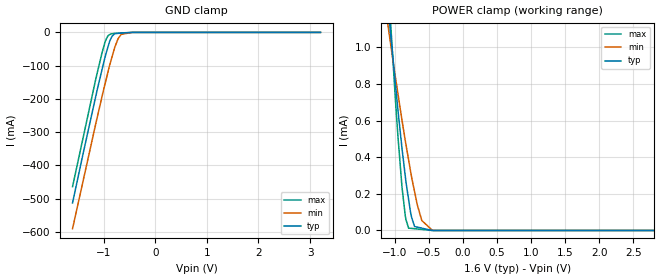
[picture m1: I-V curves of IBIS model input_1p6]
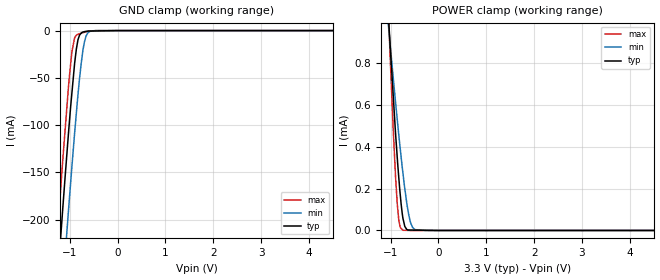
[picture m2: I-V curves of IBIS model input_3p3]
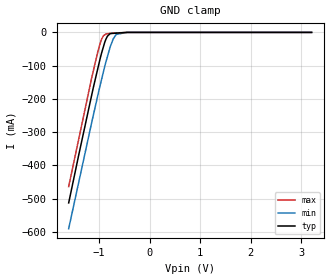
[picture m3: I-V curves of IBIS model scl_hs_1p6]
|Texas Instruments Incorporated
|Low-Power Digital Temperature Sensor with Two-Wire Interface in WCSP
| Marketing part#   Digital Voltage Range   Package-type   #pins
| TMP108YFF   1.4V - 3.6V   WCSP   6
[IBIS Ver]   4.1
[File name]   tmp108.ibs
[File Rev]   1.0
[Date]   12/13/2012
[Source]
| Texas Instruments Incorporated.
| Analog-eLab Design Center, HPA
| 12500 TI Blvd
| Dallas, TX -75243
| e-mail: elab_scm_ibis@list.ti.com
[Notes]   Revision History:
| Rev 1.0: 12/13/2012
| - Initial version of the model
| - Model generated from simulations in TISPICE
| - Model matched to SPICE simulation
| - C_comp although listed in numerical order of value are
|   obtained from varying PVT conditions. For PVT conditions for
|   each specific value refer the buffer description under
|   respective [Model]. IBIS model user is responsible for using
|   appropriate C_comp to simulate for Signal Integrity.
| - Model names with a trailing _1p6 containsthe model for 1.6V
|   [1.4V and 1.8V].Model names with a trailing _3p3 contains the
|   model for 3.3V [3.0V and 3.6V].
[Disclaimer]
| This model is designed as an aid for customers of Texas Instruments.
| TI and its licensors and suppliers make no warranties, either expressed
| or implied, with respect to this  model, including the warranties of
| merchantability or fitness for a particular purpose. The model is
| provided solely on an "as is" basis. The entire risk as to its quality
| and performance is with the customer.
[Copyright]
(C) Copyright 2012 Texas Instruments Incorporated.All rights reserved.
|   TMP108
[Component]   TMP108
[Manufacturer]   TI
[Package]   |6-WCSP
|   typ   min   max
R_pkg   0.00500   0.00500   0.00500
L_pkg   0.20000nH   0.20000nH   0.20000nH
C_pkg   0.60000pF   0.60000pF   0.60000pF
[Pin]  signal_name   model_name   R_pin   L_pin   C_pin
A1   V+   POWER   0.00500   0.20000nH  0.60000pF
A2   GND   GND   0.00500   0.20000nH  0.60000pF
B1   A0   INPUT   0.00500   0.20000nH  0.60000pF
B2   SCL   SCL   0.00500   0.20000nH  0.60000pF
C1   ALERT   ALERT   0.00500   0.20000nH  0.60000pF
C2   SDA   SDA   0.00500   0.20000nH  0.60000pF
|   Model Selectors
[Model Selector] INPUT
input_1p6  1.6V digital input
input_3p3  3.3V digital input
[Model Selector] SCL
scl_hs_1p6  1.6V digital input freq = 2.75MHz
scl_hs_3p3  3.3V digital input freq = 3.4MHz
[Model Selector] ALERT
alert_1p6  1.6V digital open-drain
alert_3p3  3.3V digital open-drain
[Model Selector] SDA
sda_fs_1p6  1.6V digital I/O_open-drain Fast_Speed freq =400KHz
sda_hs_1p6  1.6V digital I/O_open-drain High_Speed freq =3.4MHz
sda_fs_3p3  3.3V digital I/O_open-drain Fast_Speed freq =400KHz
sda_hs_3p3  3.3V digital I/O_open-drain High_Speed freq =3.4MHz
| Models and submodels in the file (10): input_1p6 (Input), input_3p3 (Input), scl_hs_1p6 (Input), scl_hs_3p3 (Input), alert_1p6 (Open_drain), alert_3p3 (Open_drain), sda_fs_1p6 (I/O_open_drain), sda_fs_3p3 (I/O_open_drain), sda_hs_1p6 (I/O_open_drain), sda_hs_3p3 (I/O_open_drain)
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|   input_1p6 Model
[Model]   input_1p6
Model_type   Input
Vinl = 0.5
Vinh = 1.4
|   typ   min   max
C_comp   3.654e-13   3.576e-13   3.663e-13
| Where nom  PVT is Nominal Process, 1.6V, 27C
|   Fast PVT is Strong Process,  1.8V, -40C
|   Slow PVT is Weak Process,   1.4V, 125C
[Voltage Range]   1.6   1.4   1.8
|Ambient Temperature   25   125   -40
|Junction Temperature
[Temperature Range]   27   125   -40
[Power Clamp Reference]   1.6   1.4   1.8
[GND Clamp Reference]   0   0   0
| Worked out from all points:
|   GND clamp passes 1 mA (typ) near -0.54 V on its own axis
|   POWER clamp passes 1 mA (typ) near -1.04 V on its own axis
[GND Clamp]
|   Voltage   I(typ)   I(min)   I(max)
-1.6V     -513.3mA   -590.8mA   -464.2mA
-1.148V   -191mA     -273.4mA   -139.1mA
-1.03V    -112.2mA   -193.3mA   -61.73mA
-979.2mV  -79.49mA   -160.3mA   -33.72mA
-912.6mV  -42.97mA   -118.3mA   -9.834mA
-884.8mV  -28.84mA   -100.7mA   -7.043mA
-835.2mV  -11.59mA   -73.39mA   -4.052mA
-778.4mV  -3.576mA   -42.89mA   -3.002mA
-718.2mV  -2.925mA   -19.01mA   -2.101mA
-659.4mV  -2.29mA    -5.982mA   -1.649mA
-449.4mV  -21.69uA   -55.42uA   -37.31uA
3.2V      0A         0A         0A
[POWER Clamp]
|   Voltage   I(typ)   I(min)   I(max)
-1.6V     3.355mA    2.44mA     4.701mA
-1.104V   1.246mA    1.136mA    1.403mA
-1.009V   880uA      887.1uA    835.4uA
-950.4mV  652uA      743.2uA    506.8uA
-891mV    444uA      598.8uA    232uA
-844.2mV  296.4uA    490.3uA    80.05uA
-795.6mV  169.6uA    385.7uA    12.84uA
-750.4mV  70.04uA    288.8uA    11.17uA
-707.2mV  21.65uA    210.4uA    9.574uA
-602mV    12.81uA    54.57uA    5.685uA
-449.4mV  0A         1.233uA    44.41nA
3.2V      0A         0A         0A
|   input_3p3 Model
[Model]   input_3p3
Model_type   Input
Vinl = 0.5
Vinh = 1.4
|   typ   min   max
C_comp   3.252e-13   3.172e-13   3.274e-13
| Where nom  PVT is Nominal Process, 3.3V, 27C
|   Fast PVT is Strong Process,  3.6V, -40C
|   Slow PVT is Weak Process,   3V, 125C
[Voltage Range]   3.3   3   3.6
|Ambient Temperature   25   125   -40
|Junction Temperature
[Temperature Range]   27   125   -40
[Power Clamp Reference]   3.3   3   3.6
[GND Clamp Reference]   0   0   0
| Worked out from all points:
|   GND clamp passes 1 mA (typ) near -0.68 V on its own axis
|   POWER clamp passes 1 mA (typ) near -1.04 V on its own axis
[GND Clamp]
|   Voltage   I(typ)   I(min)   I(max)
-3.3V     -1.779A    -1.848A    -1.738A
-1.27V    -275.6mA   -358.8mA   -225.2mA
-1.152V   -192.8mA   -275.9mA   -141.6mA
-1.099V   -156.6mA   -239.9mA   -106.9mA
-1.03V    -111mA     -193mA     -61.73mA
-954mV    -65.81mA   -143.6mA   -22.28mA
-896.4mV  -34.16mA   -107.7mA   -7.352mA
-828.3mV  -9.983mA   -68.34mA   -3.962mA
-726mV    -1.598mA   -21.55mA   -2.217mA
-624mV    -532.7uA   -2.622mA   -960.3uA
-468mV    -381uA     -82.11uA   -49.82uA
6.6V      0A         0A         0A
[POWER Clamp]
|   Voltage   I(typ)   I(min)   I(max)
-3.3V     10.7mA     7.191mA    15.83mA
-1.073V   1.122mA    1.05mA     1.21mA
-1.012V   894uA      893.9uA    845.3uA
-946.8mV  651.7uA    735.3uA    491.9uA
-896.4mV  463.8uA    612.4uA    256.6uA
-860.4mV  347.1uA    529.4uA    125.5uA
-824.4mV  240.3uA    447uA      42.46uA
-741.6mV  57.86uA    273.2uA    1.007uA
-702.9mV  19.11uA    199.7uA    771.7nA
-618mV    2.222uA    71.78uA    255.7nA
-492mV    1.767uA    4.112uA    0A
6.6V      0A         0A         0A
|   scl_hs_1p6 Model
[Model]   scl_hs_1p6
Model_type   Input
Vinl = 0.5
Vinh = 1.4
|   typ   min   max
C_comp   2.996e-13   2.983e-13   3.022e-13
| Where nom  PVT is Nominal Process, 1.6V, 27C
|   Fast PVT is Strong Process,  1.8V, -40C
|   Slow PVT is Weak Process,   1.4V, 125C
[Voltage Range]   1.6   1.4   1.8
|Ambient Temperature   25   125   -40
|Junction Temperature
[Temperature Range]   27   125   -40
[Power Clamp Reference]   1.6   1.4   1.8
[GND Clamp Reference]   0   0   0
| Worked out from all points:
|   GND clamp passes 1 mA (typ) near -0.54 V on its own axis
[GND Clamp]
|   Voltage   I(typ)   I(min)   I(max)
-1.6V     -513.3mA   -590.8mA   -464.2mA
-1.148V   -191mA     -273.4mA   -139.1mA
-1.03V    -112.2mA   -193.3mA   -61.73mA
-979.2mV  -79.49mA   -160.3mA   -33.72mA
-912.6mV  -42.97mA   -118.3mA   -9.834mA
-884.8mV  -28.84mA   -100.7mA   -7.043mA
-835.2mV  -11.59mA   -73.4mA    -4.052mA
-778.4mV  -3.576mA   -42.89mA   -3.002mA
-718.2mV  -2.925mA   -19.01mA   -2.101mA
-659.4mV  -2.29mA    -5.984mA   -1.649mA
-449.4mV  -21.69uA   -55.96uA   -37.31uA
3.2V      0A         0A         0A
[POWER Clamp]
|   Voltage   I(typ)   I(min)   I(max)
-1.6V     0A         0A         0A
-1.598V   0A         0A         0A
3.2V      0A         0A         0A
